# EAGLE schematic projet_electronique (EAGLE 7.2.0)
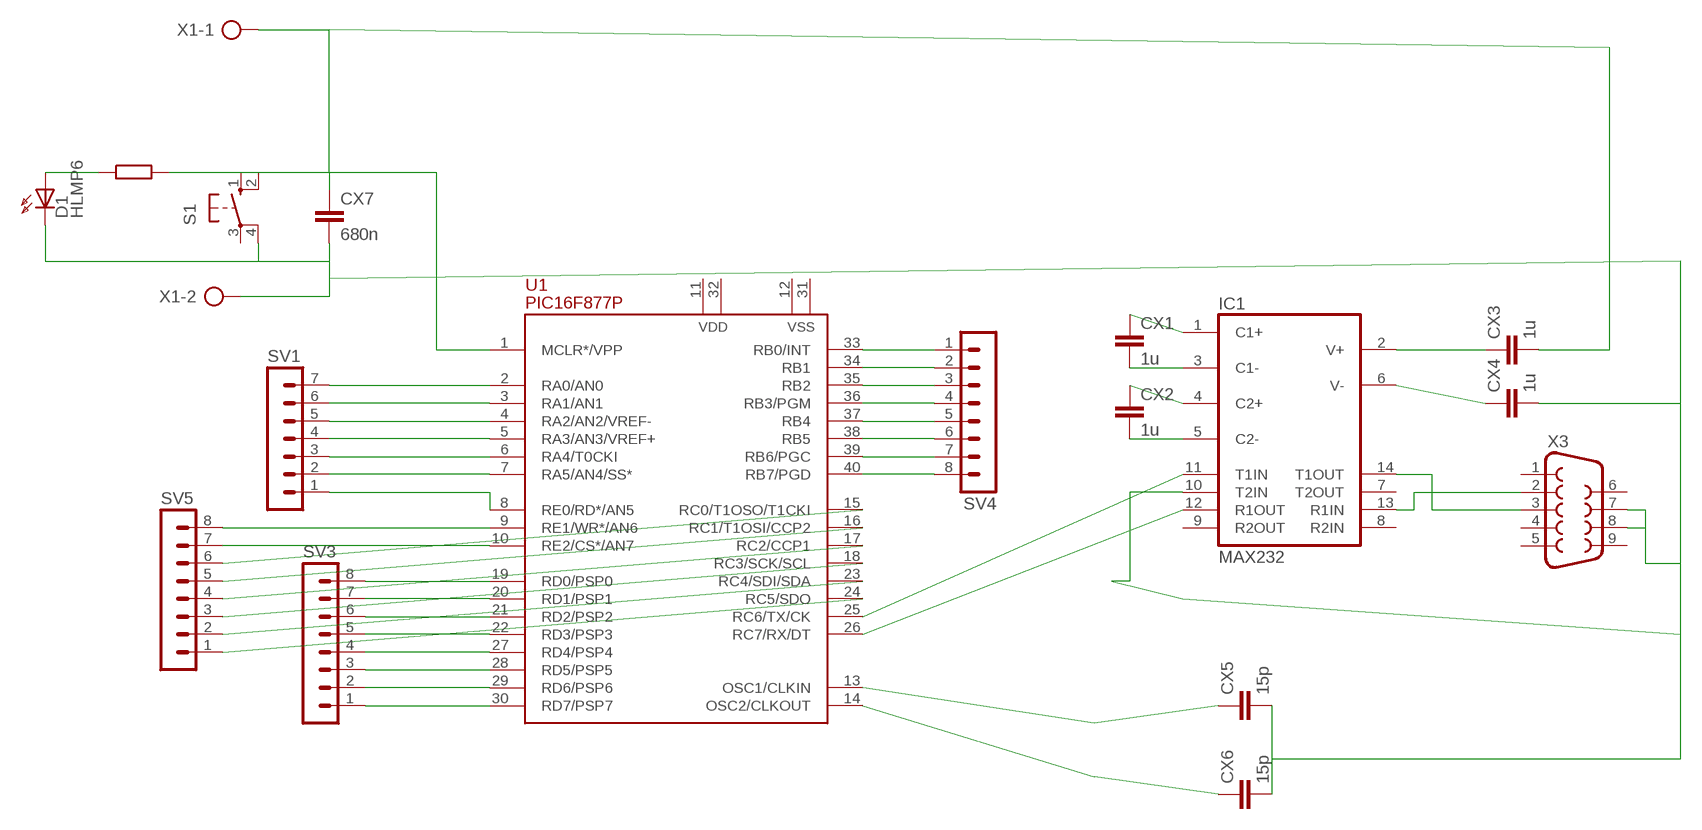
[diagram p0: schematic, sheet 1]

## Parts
CX1  1u  CXXC10B5  [XC10B5]
CX2  1u  CXXC10B5  [XC10B5]
CX3  1u  CXXC10B5  [XC10B5]
CX4  1u  CXXC10B5  [XC10B5]
CX5  15p  CXXC10B5  [XC10B5]
CX6  15p  CXXC10B5  [XC10B5]
CX7  680n  CXXC10B5  [XC10B5]
D1  HLMP6  [HLMP6]
IC1  MAX232  [DIL16]
S1  10-XX  [B3F-10XX]
SV1  MA07-1  [MA07-1]
SV3  MA08-1  [MA08-1]
SV4  MA08-1  [MA08-1]
SV5  MA08-1  [MA08-1]
U1  PIC16F877P  [DIL40]
X1  AK500/2-H  [AK500/2-H]
X3  F09V  [F09V]

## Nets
N$1: D1.A
N$2: CX3.2 CX7.1 S1.2(S1) U1.1(MCLR*/VPP) X1.1
N$3: CX4.2 CX5.2 CX6.2 CX7.2 D1.K IC1.10(T2IN) S1.4(P1) X1.2 X3.7 X3.8
N$4: CX5.1 U1.13(OSC1/CLKIN)
N$5: CX1.1 IC1.1(C1+)
N$7: CX6.1 U1.14(OSC2/CLKOUT)
N$8: CX1.2 IC1.3(C1-)
N$9: CX2.1 IC1.4(C2+)
N$10: CX2.2 IC1.5(C2-)
N$11: CX3.1 IC1.2(V+)
N$12: CX4.1 IC1.6(V-)
N$13: IC1.11(T1IN) U1.25(RC6/TX/CK)
N$14: IC1.12(R1OUT) U1.26(RC7/RX/DT)
N$15: SV1.7 U1.2(RA0/AN0)
N$16: IC1.14(T1OUT) X3.3
N$17: IC1.13(R1IN) X3.2
N$18: SV4.1 U1.33(RB0/INT)
N$19: SV4.2 U1.34(RB1)
N$20: SV4.3 U1.35(RB2)
N$21: SV4.4 U1.36(RB3/PGM)
N$22: SV1.6 U1.3(RA1/AN1)
N$23: SV1.5 U1.4(RA2/AN2/VREF-)
N$24: SV1.4 U1.5(RA3/AN3/VREF+)
N$25: SV1.3 U1.6(RA4/T0CKI)
N$26: SV1.2 U1.7(RA5/AN4/SS*)
N$27: SV1.1 U1.8(RE0/RD*/AN5)
N$28: SV3.8 U1.19(RD0/PSP0)
N$29: SV3.7 U1.20(RD1/PSP1)
N$30: SV3.6 U1.21(RD2/PSP2)
N$31: SV3.5 U1.22(RD3/PSP3)
N$32: SV3.4 U1.27(RD4/PSP4)
N$33: SV3.3 U1.28(RD5/PSP5)
N$34: SV3.2 U1.29(RD6/PSP6)
N$35: SV3.1 U1.30(RD7/PSP7)
N$36: SV4.5 U1.37(RB4)
N$37: SV4.6 U1.38(RB5)
N$38: SV4.7 U1.39(RB6/PGC)
N$39: SV4.8 U1.40(RB7/PGD)
N$40: SV5.8 U1.9(RE1/WR*/AN6)
N$41: SV5.7 U1.10(RE2/CS*/AN7)
N$42: SV5.6 U1.15(RC0/T1OSO/T1CKI)
N$43: SV5.5 U1.16(RC1/T1OSI/CCP2)
N$44: SV5.4 U1.17(RC2/CCP1)
N$45: SV5.3 U1.18(RC3/SCK/SCL)
N$46: SV5.2 U1.23(RC4/SDI/SDA)
N$47: SV5.1 U1.24(RC5/SDO)
Unconnected: IC1.7(T2OUT) IC1.8(R2IN) IC1.9(R2OUT) S1.1(S) S1.3(P) U1.11(VDD) U1.12(VSS) U1.31(VSS) U1.32(VDD) X3.1 X3.4 X3.5 X3.6 X3.9

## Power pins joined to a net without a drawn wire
GND: IC1.15(GND)
VCC: IC1.16(VCC)

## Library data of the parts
CX1-CX7 = rcl:CX: X CAPACITOR
D1 = display-hp:HLMP6: LED; MF: AGILENT TECHNOLOGIES; MPN: HLMP-6500; OC_FARNELL: 1652490; OC_NEWARK: 40K0088
IC1 = maxim:MAX232: RS232 TRANSCEIVER; MF: MAXIM; MPN: MAX232ACPE+; OC_FARNELL: 9723773; OC_NEWARK: 68K4544
S1 = switch-omron:10-XX: OMRON SWITCH; MPN: B3F-1000; OC_FARNELL: 176432; OC_NEWARK: 36M3542
SV1 = con-lstb:MA07-1: PIN HEADER; OC_FARNELL: unknown; OC_NEWARK: unknown
SV3-SV5 = con-lstb:MA08-1: PIN HEADER; OC_FARNELL: unknown; OC_NEWARK: unknown
U1 = pic16f87x:PIC16F877: FLASH MICROCONTROLLER
X1 = con-ptr500:AK500/2-H: CONNECTOR; OC_FARNELL: unknown; OC_NEWARK: unknown
X3 = con-subd:F09: SUB-D; OC_FARNELL: unknown; OC_NEWARK: unknown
